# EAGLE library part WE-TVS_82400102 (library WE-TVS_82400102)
TVS Diode Array WE-TVS, High Speed Series - Low capazity - No leakage current - Low clamping voltage - high ESD voltage protection -- USB 1.0 - 2.0 Flow Thru Design
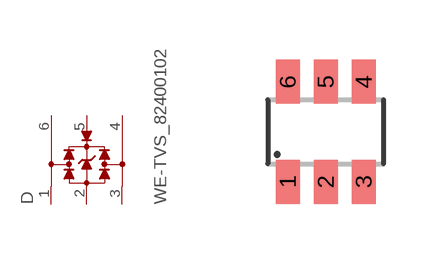
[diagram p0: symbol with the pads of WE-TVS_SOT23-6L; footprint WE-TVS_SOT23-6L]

Designator prefix D

## WE-TVS_82400102 (MPN: 82400102; OC_FARNELL: 1825875; OC_NEWARK: 79R6945; PACKAGE: SOT23-6L; SUPPLIER: Wuerth Elektronik)  [WE-TVS_SOT23-6L]
1  1  pas
2  GND  pwr
3  2  pas
4  3  pas
5  VDD  pwr
6  4  pas

## Footprint WE-TVS_SOT23-6L (pad centres in mm)
TVS Diode Array WE-TVS
smd 0.6 x 1.1: 1 -0.95,-1.25; 2 0,-1.25; 3 0.95,-1.25; 4 0.95,1.25; 5 0,1.25; 6 -0.95,1.25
